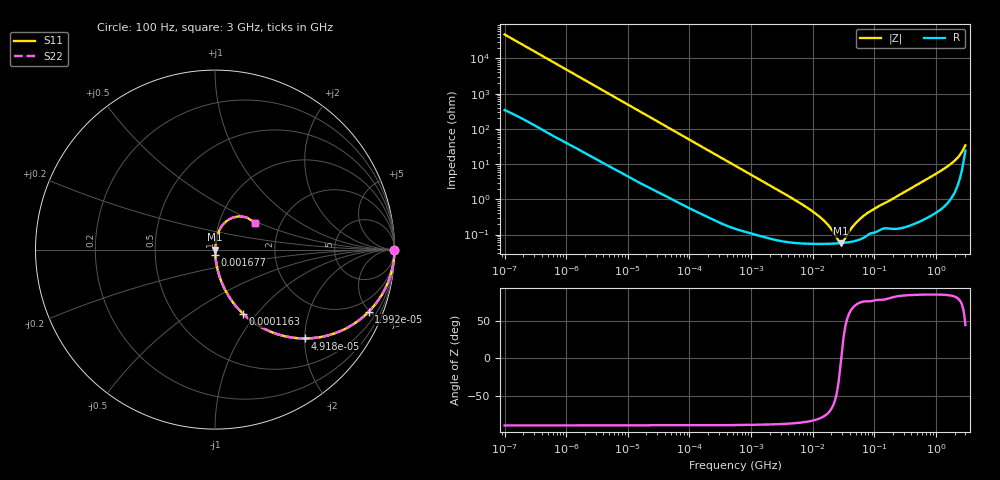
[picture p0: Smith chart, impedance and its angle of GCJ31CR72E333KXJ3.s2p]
!Murata Part Number: GCJ31CR72E333KXJ3
!These Parameters are Measured in Series Mode Connection
!Data Generated on Mar 13, 2026
!  o--ll--o
!Port1  Port2
!  o------o
!Operation Temp=25[degC], DC Bias Voltage=0[V]
!Freq. Start=100[Hz] Stop=3[GHz] 401[Steps]
# Hz S RI R 50
!Freq.(Hz) S11(Real) S11(Imag) S21(Real) S21(Imag) S12(Real) S12(Imag) S22(Real) S22(Imag)
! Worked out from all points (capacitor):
!   401 points, 100 Hz to 3 GHz, reference 50 ohm
!   read as one part in series: C = 33.4 nF near 109 Hz
!   lowest |Z| = 57.2 mohm at 28.73 MHz (marker M1)
!   series resonance near 28.96 MHz, so ESL is about 910 pH
!   S11 on the Smith chart (normalised r, x): 100 Hz: open; 19.92 kHz: 1.05, -4.93; 49.18 kHz: 1.02, -2.01; 116.3 kHz: 1.01, -0.85; 1.677 MHz: 1.00, -0.06; 3 GHz: 1.48, +0.48
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100  1 -0.0021  1.94e-05 0.0021  1.94e-05 0.0021  1 -0.0021
1788  0.9983 -0.0369  0.00168 0.0369  0.00168 0.0369  0.9983 -0.0369
6790  0.9798 -0.1363  0.0202 0.1363  0.0202 0.1363  0.9798 -0.1363
19917  0.8561 -0.3462  0.1439 0.3462  0.1439 0.3462  0.8561 -0.3462
31977  0.7012 -0.4527  0.2988 0.4527  0.2988 0.4527  0.7012 -0.4527
49177  0.5016 -0.4948  0.4984 0.4948  0.4984 0.4948  0.5016 -0.4948
116311  0.1568 -0.3579  0.8432 0.3579  0.8432 0.3579  0.1568 -0.3579
221826  0.0505 -0.2127  0.9495 0.2127  0.9495 0.2127  0.0505 -0.2127
547723  0.00972 -0.0904  0.9903 0.0904  0.9903 0.0904  0.00972 -0.0904
1677156  0.00174 -0.03  0.9983 0.03  0.9983 0.03  0.00174 -0.03
9794414  0.000566 -0.0046  0.9994 0.0046  0.9994 0.0046  0.000566 -0.0046
1.713898e7  0.000549 -0.00193  0.9995 0.00193  0.9995 0.00193  0.000549 -0.00193
2.635803e7  0.000565 -0.000331  0.9994 0.000331  0.9994 0.000331  0.000565 -0.000331
2.872754e7  0.000571 -2.83e-05  0.9994 2.83e-05  0.9994 2.83e-05  0.000571 -2.83e-05
3.131008e7  0.00058 0.000274  0.9994 -0.000274  0.9994 -0.000274  0.00058 0.000274
4.612319e7  0.000647 0.00169  0.9994 -0.00169  0.9994 -0.00169  0.000647 0.00169
6.234031e7  0.000769 0.00296  0.9992 -0.00296  0.9992 -0.00296  0.000769 0.00296
1.751444e8  0.00156 0.009  0.9984 -0.009  0.9984 -0.009  0.00156 0.009
1.022825e9  0.00714 0.0536  0.9929 -0.0536  0.9929 -0.0536  0.00714 0.0536
1.868531e9  0.024 0.1072  0.976 -0.1072  0.976 -0.1072  0.024 0.1072
2.419119e9  0.0621 0.1572  0.9379 -0.1572  0.9379 -0.1572  0.0621 0.1572
3e9  0.2237 0.1499  0.7763 -0.1499  0.7763 -0.1499  0.2237 0.1499
